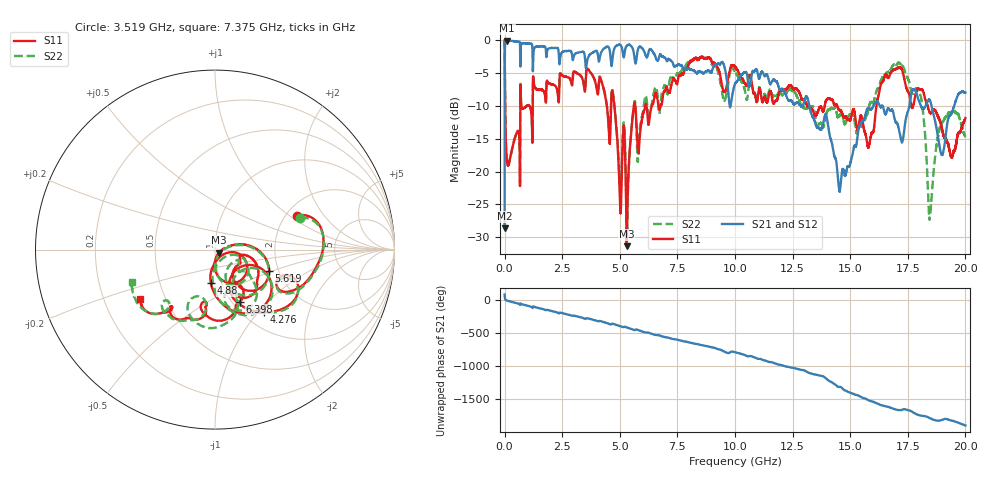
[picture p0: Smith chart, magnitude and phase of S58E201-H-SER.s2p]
!{S58E201}
!Johanson Technology Inc.
!www.johansontechnology.com
!Test Board Conditions:
!Substrate Type  RO4350B
!Substrate Thickness  60 mil
!Substrate Dk  3.66
!TL Type: GCPW
!TL Trace Width  115 mil
!TL Gap  52 mil
!Electrode orientation  Horizontal
!DUT TOPOLOGY	SERIES
!Mounting Pad LxW  55x428 mil
! Created Wed Apr 14 11:28:37 2021
# mhz S ma R 50
! 2 Port Network Data from SP1.SP block
! freq  magS11  angS11  magS21  angS21  magS12  angS12  magS22  angS22
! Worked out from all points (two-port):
!   20001 points, 300 kHz to 20 GHz, reference 50 ohm
!   highest |S21| = -0.07 dB at 107.3 MHz (marker M1); lowest = -28.7 dB at 300 kHz (marker M2)
!   |S21| within 3 dB of the highest: 1.24 GHz to 2.366 GHz (1.125 GHz wide, 62.4 % of centre); 2.401 GHz to 3.496 GHz (1.094 GHz wide, 37.1 % of centre)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
!   lowest |S11| = -31.4 dB at 5.301 GHz (marker M3), VSWR 1.06, Z = 52.1 - j1.81 ohm
!   |S11| at or under -10 dB: 4.763 GHz to 5.612 GHz (848.6 MHz wide, 16.4 % of centre); 14.44 GHz to 16.14 GHz (1.697 GHz wide, 11.1 % of centre); 18.36 GHz to end of sweep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
!   |S22| runs from -29.7 to 0.0 dB; largest |S21 - S12| = 0.0098
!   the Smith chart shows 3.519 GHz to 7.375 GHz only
!   S11 on the Smith chart (normalised r, x): 3.519 GHz: 2.30, +1.15; 4.276 GHz: 1.23, -1.07; 4.88 GHz: 0.89, -0.34; 5.619 GHz: 1.78, -0.47; 6.398 GHz: 1.09, -0.70; 7.375 GHz: 0.36, -0.26
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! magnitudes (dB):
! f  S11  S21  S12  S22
! 300 kHz  0.0  -28.7  -28.7  0.0
! 107.3 MHz  -18.7  -0.1  -0.1  -18.6
! 1.323 GHz  -7.3  -1.1  -1.1  -7.3
! 3.334 GHz  -5.5  -1.8  -1.8  -5.6
! 3.519 GHz  -6.1  -4.1  -4.1  -5.9
! 4.276 GHz  -7.1  -1.4  -1.4  -7.1
! 4.88 GHz  -14.6  -0.8  -0.8  -14.2
! 5.301 GHz  -31.4  -0.9  -0.9  -28.5
! 5.619 GHz  -9.8  -2.1  -2.2  -9.8
! 6.398 GHz  -9.9  -1.6  -1.6  -9.5
! 6.667 GHz  -9.8  -3.1  -3.1  -9.4
! 7.375 GHz  -6.0  -4.1  -4.1  -6.1
! 10 GHz  -4.0  -6.7  -6.6  -4.7
! 13.33 GHz  -10.6  -11.4  -11.6  -10.1
! 13.97 GHz  -9.1  -11.6  -11.6  -11.1
! 14.55 GHz  -10.6  -23.1  -22.9  -11.5
! 15.8 GHz  -16.2  -10.3  -10.4  -10.2
! 16.67 GHz  -5.6  -10.4  -10.6  -4.8
! 18.02 GHz  -7.5  -9.6  -9.6  -8.1
! 18.47 GHz  -11.1  -9.2  -9.2  -26.8
! 18.99 GHz  -13.6  -17.5  -17.4  -12.6
! 20 GHz  -11.8  -8.0  -8.0  -14.7
